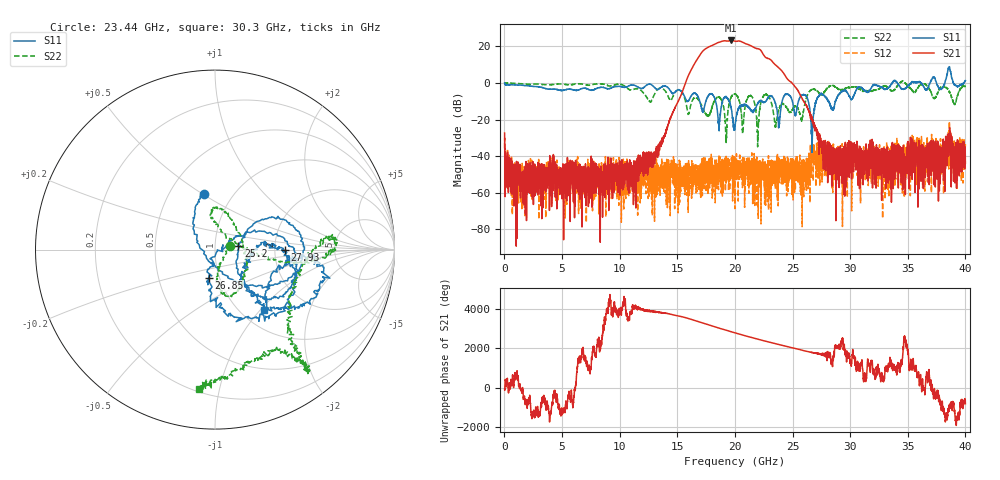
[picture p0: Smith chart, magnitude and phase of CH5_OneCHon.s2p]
!Keysight Technologies,N5245B,MY57181321,A.14.80.03
!Date: Thursday, March 28, 2024 18:49:48
!Correction: S11(C  2-Port  )
!S21(C  2-Port  )
!S12(C  2-Port  )
!S22(C  2-Port  )
!S2P File: Measurements: S11, S21, S12, S22:
# Hz S  RI  R 50
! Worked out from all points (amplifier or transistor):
!   4000 points, 10 MHz to 40 GHz, reference 50 ohm
!   highest |S21| = 23.2 dB at 19.69 GHz (marker M1)
!   |S21| within 3 dB of that: 17.91 GHz to 21.42 GHz (3.507 GHz wide, 17.8 % of centre)
!   unconditionally stable (mu >= 1): 19.86 MHz to 33.64 GHz; 36.2 GHz to 36.93 GHz; 38.95 GHz to 39.87 GHz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
!   at 6.67 GHz: K = 3601.27, MAG = -43.2 dB, |S12| = -46.0 dB
!   at 20.01 GHz: K = 5.65, MAG = 24.0 dB, |S12| = -46.3 dB
!   at 40 GHz: K = -446.40, MSG = -5.2 dB, |S12| = -33.4 dB
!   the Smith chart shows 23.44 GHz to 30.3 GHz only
!   S11 on the Smith chart (normalised r, x): 23.44 GHz: 0.73, +0.51; 25.2 GHz: 1.30, +0.06; 26.85 GHz: 0.89, -0.29; 27.93 GHz: 2.27, -0.02; 30.3 GHz: 1.26, -1.05
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1e7  1.002 -0.0595  0.0248 -0.0349  0.00791 0.0141  -0.9767 0.0249
6.68e9  0.5039 0.4697  -0.000945 0.000372  -0.00173 -0.00192  0.9346 0.0901
1.334e10  -0.5992 -0.2767  -0.0103 -0.013  -0.000476 0.00349  -0.6822 -0.0756
1.707e10  0.1904 0.1256  2.062 6.128  0.00252 -0.00261  0.1074 0.2298
1.752e10  0.2626 -0.2317  8.477 -2.548  -0.0027 -0.00654  -0.1257 0.0475
1.798e10  0.4862 -0.1382  -1.701 -10.23  -0.00319 -0.00411  0.0574 -0.1983
1.848e10  0.1638 0.0173  -12.26 1.894  -0.00395 -0.00203  0.3847 -0.137
1.897e10  -0.0803 -0.3486  1.193 13.93  0.00566 -0.00486  0.2498 0.0399
1.969e10  0.1813 -0.0739  10.97 -9.322  0.00403 0.00352  -0.2784 -0.3247
2.001e10  -0.0381 0.0556  -0.9931 -13.64  -0.0048 0.000759  -0.2132 -0.4507
2.049e10  -0.0952 -0.205  -13.55 -1.951  0.00383 -0.00149  -0.0233 -0.2162
2.098e10  0.2263 -0.1043  -2.398 11.33  0.0022 -0.002  -0.1599 0.2596
2.153e10  -0.065 0.1496  9.295 2.986  -0.00143 0.00262  -0.3197 0.2309
2.209e10  -0.1723 -0.2604  2.269 -8.099  0.00139 0.00383  0.1296 0.0151
2.344e10  -0.0631 0.3097  0.1992 3.251  0.00187 0.000981  0.084 0.0217
2.52e10  0.1298 0.0226  -0.7618 -0.221  -0.00579 0.00458  0.0287 0.2285
2.667e10  0.0431 -0.011  0.1182 -0.0248  0.00195 0.00772  0.6546 0.00201
2.685e10  -0.0352 -0.1566  0.0617 -0.0382  -0.00448 -0.00631  0.6623 0.0615
2.793e10  0.3881 -0.00396  0.00158 -0.0184  -0.00245 0.00156  0.4238 -0.5056
3.03e10  0.2717 -0.338  -0.00232 0.00826  0.00251 -0.00755  -0.09 -0.7783
3.334e10  0.1709 -0.7193  -0.00873 0.00213  -0.00093 0.00431  -0.3328 -0.6338
4e10  -0.8592 -0.7743  -0.000974 -0.00632  0.0211 -0.00317  0.4875 0.6338
